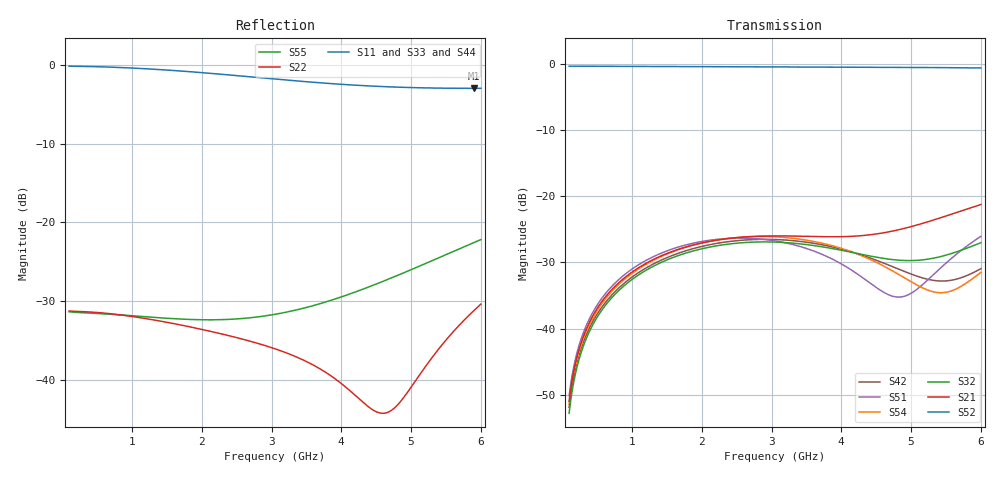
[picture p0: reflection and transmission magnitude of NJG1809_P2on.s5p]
! Port1:P1  Port2:P2  Port3:P3  Port4:P4  Port5:PC
# hz S ma R 50
! 5 Port Network Data from SP1.SP block
! freq  magS11  angS11  magS12  angS12  magS13  angS13  magS14  angS14
!  magS15  angS15
!  magS21  angS21  magS22  angS22  magS23  angS23
!  magS24  angS24  magS25  angS25
!  magS31  angS31  magS32  angS32
!  magS33  angS33  magS34  angS34  magS35  angS35
!  magS41  angS41
!  magS42  angS42  magS43  angS43  magS44  angS44  magS45  angS45
!  magS51  angS51  magS52  angS52  magS53  angS53  magS54  angS54
!  magS55  angS55
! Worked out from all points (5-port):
!   591 points, 100 MHz to 6 GHz, reference 50 ohm
!   strongest paths, dB at 100 MHz, 1.57 GHz, 3.05 GHz, 4.53 GHz, 6 GHz:
!     S52: -0.4, -0.4, -0.5, -0.5, -0.6
!     S21: -51.0, -28.4, -26.0, -25.7, -21.3
!     S32: -52.8, -29.3, -26.9, -29.3, -27.0
!     S54: -51.5, -28.5, -26.1, -30.1, -31.5
!     S51: -50.1, -28.0, -26.8, -34.0, -26.1
!     S42: -51.9, -29.0, -26.5, -29.8, -31.0
!   lowest |S11| = -3.0 dB at 5.9 GHz (marker M1), VSWR 5.86, Z = 11.6 + j29.2 ohm
!   |S11| at or under -10 dB: nowhere
